PROGRAM MAIN
VAR
	AODB		: ARRAY[0..1] OF ST_IEC870_5_101AODBEntry;(* Application object database including 2 data points *)
	hTable		: T_HAODBTable;(* Application object database handle *)
	fbClient	: FB_IEC870_5_104Master;(* IEC 60870-5-104 master function block instance *)

	nCAA		: DWORD := 7;(* Common ASDU address of remote (slave) station *)

	bSPI		AT%MX0.0 : BOOL;(* Single point information (data point used in monitoring direction slave->master) *)
	bSCS		AT%MX1.5 : BOOL;(* Single command state (data point used in control direction master->slave) *)

	fbCloseAll	: FB_SocketCloseAll;(* Closes all opened sockets after PLC reset or new PLC project download *)
	bInit		: BOOL := TRUE;
	nInitErr	: UDINT;
END_VAR

fbCloseAll( bExecute := bInit );
IF fbCloseAll.bBusy AND NOT bInit THEN
	RETURN;
END_IF

IF bInit THEN
	bInit := FALSE;

	(* Configure protocol parameter *)
	fbClient.protPara.sRemoteHost := '127.0.0.1';(* IP address of remote (slave) station *)
	fbClient.protPara.nRemotePort := 2404;(* Port number (default) of remote (slave) station *)

	(* Configure system parameter *)
	fbClient.sysPara.asduAddr := nCAA;(* Common ASDU address of remote (slave) station *)
	fbClient.sysPara.dbgMode := IEC870_DEBUGMODE_DEVSTATE(* OR IEC870_DEBUGMODE_LINKERROR OR IEC870_DEBUGMODE_ASDU OR IEC870_DEBUGMODE_LINKLAYER *);(* Enable debug output of device state change *)


	nInitErr := F_iecCreateTableHnd( ADR( AODB ), SIZEOF( AODB ), hTable );(* Initialize database handle *)


	(* Configure one single point in monitoring direction *)
	nInitErr := F_iecAddTableEntry( M_SP_NA_1,(* Type is single point *)
									nCAA,(* Common ASDU address *)
									100,(* Information object address *)
									IEC870_GRP_INROGEN,(* Interrogation group *)
									0,(* Multiplier (not used) *)
									MAP_AREA_MEMORY,(* Map this single point value TO PLC memory area (buffer) *)
									0,(* Map TO byte offset *)
									0,(* Map TO bit offset *)
									0,(* Not used *)
									hTable );(* Application object database handle *)

	(* Configure one single command in control direction *)
	nInitErr := F_iecAddTableEntry( C_SC_NA_1,(* Type is single command *)
									nCAA,(* Common ASDU address *)
									10,(* Information object address *)
									0,(* Group (not used) *)
									0,(* Multiplier (not used) *)
									MAP_AREA_MEMORY, (* Map this single command value FROM PLC memory area (buffer) *)
									1,(* Map FROM byte offset *)
									5,(* Map FROM bit offset *)
									0,(* Not used *)
									hTable );(* Application object database handle *)

ELSE
	fbClient(	pAOEntries	:= ADR( AODB ),(* Start address of application object database *)
				cbAOEntries := SIZEOF( AODB ),(* Byte size of application object database *)
				pInputs 	:= 0,(* Not used *)
				cbInputs 	:= 0,(* Not used *)
				pOutputs 	:= 0,(* Not used *)
				cbOutputs 	:= 0,(* Not used *)
				pMemory 	:= ADR( %MB0 ),(* Start address of memory area (buffer). Memory buffer where the data point values are mapped to and from *)
				cbMemory 	:= 2,(* Byte size of memory area (buffer) = 2 byte (%MB0..%MB1) *)
				pData 		:= 0,(* Not used *)
				cbData 		:= 0,(* Not used *)
				hTable 		:= hTable,(* Application object database handle *)
				bEnable 	:= TRUE(* Enable communication *) );


	(* Check for device errors, remove them and log errror message to the TwinCAT->Error List CTRL+^, E *)
	REPEAT
		fbClient.system.device.errors.RemoveError( );
		IF fbClient.system.device.errors.bOk THEN
			ADSLOGSTR( ADSLOG_MSGTYPE_ERROR OR ADSLOG_MSGTYPE_LOG, 'IEC60870-5-104 master error: 0x%s',
						DWORD_TO_HEXSTR( fbClient.system.device.errors.getError.nErrId, 8, FALSE) );
		END_IF
	UNTIL NOT fbClient.system.device.errors.bOk
	END_REPEAT

END_IF

END_PROGRAM
